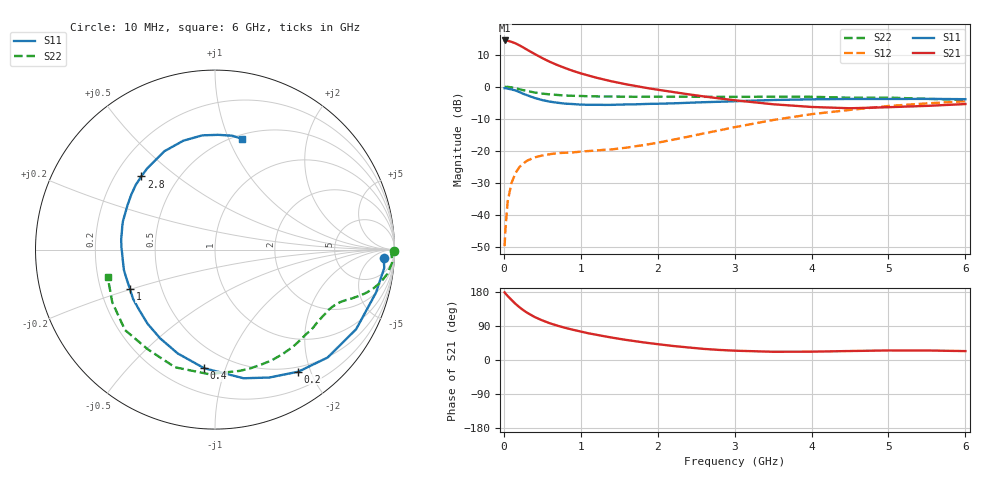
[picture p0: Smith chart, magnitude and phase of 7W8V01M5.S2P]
! Infineon Technologies  Discrete & RF Semiconductors
! BFS17W
! Si NPN RF Bipolar Junction Transistor in SOT323
! VCE = 8 V  IC = 1.5 mA
! Common Emitter S-Parameters:  August  1999
# GHz  S  MA  R  50
!  f  S11  S21  S12  S22
! GHz  MAG  ANG  MAG  ANG  MAG  ANG  MAG  ANG
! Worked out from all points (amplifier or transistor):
!   36 points, 10 MHz to 6 GHz, reference 50 ohm
!   highest |S21| = 14.4 dB at 10 MHz (marker M1)
!   |S21| within 3 dB of that: start of sweep to 310 MHz
!   unconditionally stable (mu >= 1): 944.1 MHz to 2.93 GHz; 4.222 GHz to end of sweep
!   at 250 MHz: K = 0.30, MSG = 18.2 dB, |S12| = -24.1 dB
!   at 1.4 GHz: K = 1.26, MAG = 7.6 dB, |S12| = -19.7 dB
!   at 6 GHz: K = 1.08, MAG = -2.2 dB, |S12| = -4.6 dB
!   S11 on the Smith chart (normalised r, x): 10 MHz: 19, -16; 200 MHz: 0.43, -1.81; 400 MHz: 0.36, -0.85; 1 GHz: 0.33, -0.20; 2.8 GHz: 0.31, +0.38; 6 GHz: 0.54, +1.12
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0.01  0.9412 -2.9  5.258 178.4  0.0032 84.9  0.9999 -0.3
0.02  0.9485 -6.2  5.231 175.6  0.0058 88.6  0.9835 -1.5
0.05  0.9284 -15.0  5.204 168.9  0.0161 83.8  0.9901 -4.1
0.1  0.9028 -29.4  4.994 158.6  0.0312 73.8  0.9708 -7.9
0.15  0.869 -43.8  4.751 148.5  0.044 66.5  0.9417 -11.1
0.2  0.8234 -55.7  4.428 139.8  0.0547 61.3  0.9108 -13.6
0.25  0.7744 -67.0  4.101 132.0  0.0623 55.4  0.8803 -15.7
0.3  0.7341 -77.5  3.781 125.1  0.0692 51.3  0.8535 -17.3
0.4  0.6637 -95.2  3.234 113.5  0.0782 45.6  0.8083 -19.7
0.5  0.6146 -109.8  2.786 104.5  0.0836 42.5  0.7761 -21.4
0.6  0.581 -121.8  2.43 96.8  0.0877 40.3  0.7547 -22.9
0.7  0.5583 -132.3  2.16 90.4  0.0912 39.4  0.7385 -24.5
0.8  0.5405 -141.0  1.942 84.7  0.0924 39.6  0.7259 -26.2
1  0.5222 -155.2  1.609 75.1  0.0961 41.1  0.7126 -29.6
1.1  0.5189 -162.2  1.488 70.5  0.0983 42.8  0.7061 -31.7
1.6  0.5261 173.5  1.079 52.7  0.1112 53.0  0.693 -42.5
2.2  0.547 152.9  0.822 37.0  0.1477 65.3  0.6933 -57.3
2.8  0.5785 135.2  0.653 26.6  0.2068 70.1  0.6903 -73.4
3.5  0.6164 117.2  0.529 21.7  0.3 68.1  0.6946 -92.9
4.5  0.6405 96.3  0.458 23.7  0.4317 56.1  0.6697 -124.0
5.5  0.6419 81.5  0.499 25.1  0.546 42.3  0.6431 -152.9
6  0.6353 76.2  0.533 23.5  0.5896 35.7  0.617 -165.8
